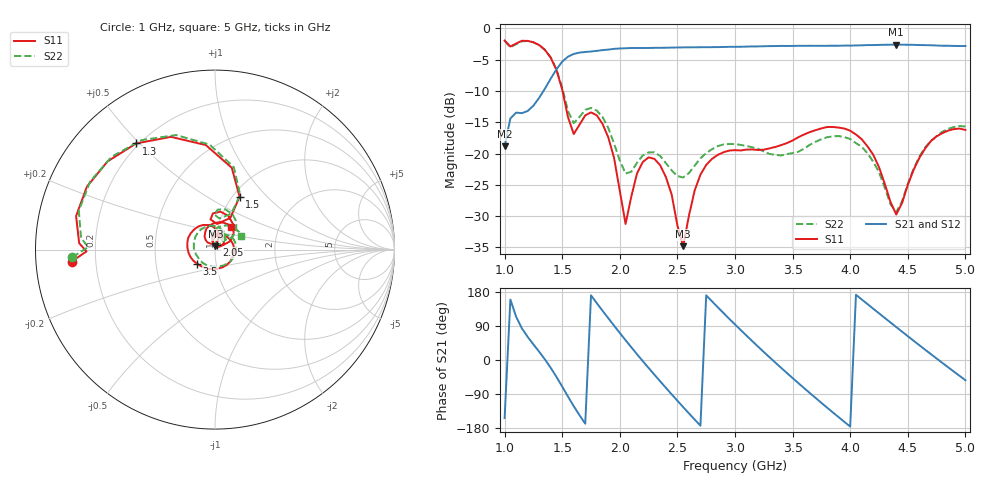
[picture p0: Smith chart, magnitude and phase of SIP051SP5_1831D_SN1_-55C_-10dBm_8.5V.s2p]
# GHz  S  dB  R  50
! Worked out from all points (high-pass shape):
!   81 points, 1 GHz to 5 GHz, reference 50 ohm
!   highest |S21| = -2.60 dB at 4.4 GHz (marker M1); lowest = -18.8 dB at 1 GHz (marker M2)
!   |S21| within 3 dB of the highest: 1.488 GHz to end of sweep
!   lowest |S11| = -34.8 dB at 2.55 GHz (marker M3), VSWR 1.04, Z = 50.2 + j1.82 ohm
!   |S11| at or under -10 dB: 1.503 GHz to end of sweep
!   |S22| runs from -29.4 to -2.0 dB; largest |S21 - S12| = 0.0021
!   S11 on the Smith chart (normalised r, x): 1 GHz: 0.11, -0.04; 1.3 GHz: 0.19, +0.49; 1.5 GHz: 1.08, +0.71; 2.05 GHz: 1.02, +0.05; 3.5 GHz: 0.81, -0.13; 5 GHz: 1.16, +0.30
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1  -1.93 -175.2  -18.83 -153.3  -18.81 -153.1  -1.98 -176.9
1.1  -2.41 177.3  -13.46 114.1  -13.45 114.0  -2.51 175.1
1.3  -2.65 126.6  -11.09 21.9  -11.10 21.7  -2.68 123.9
1.5  -9.76 65.1  -5.32 -70.1  -5.31 -70.1  -9.47 65.3
1.6  -16.87 85.6  -4.08 -121.8  -4.07 -121.7  -15.14 82.1
1.7  -13.89 93.3  -3.76 -168.1  -3.77 -168.0  -13.01 86.0
1.9  -17.40 39.9  -3.38 110.3  -3.37 110.4  -15.90 42.4
2.05  -31.24 72.2  -3.17 52.3  -3.17 52.3  -23.19 51.3
2.2  -21.33 91.7  -3.13 -3.1  -3.13 -3.1  -20.29 67.8
2.35  -21.85 52.2  -3.10 -56.1  -3.10 -56.0  -20.37 48.4
2.55  -34.79 83.7  -3.03 -124.2  -3.03 -124.2  -23.81 53.5
2.75  -21.81 79.3  -3.01 170.6  -3.01 170.7  -19.91 53.8
3  -19.45 -2.3  -2.94 93.8  -2.94 93.8  -18.49 10.8
3.25  -19.37 -81.6  -2.85 21.2  -2.86 21.2  -19.65 -48.5
3.5  -17.91 -141.9  -2.80 -47.7  -2.79 -47.7  -19.93 -132.5
3.7  -16.25 176.3  -2.79 -100.2  -2.79 -100.2  -18.10 161.6
4  -16.35 115.6  -2.75 -175.7  -2.75 -175.7  -17.67 86.9
4.15  -18.83 86.8  -2.67 147.6  -2.67 147.5  -19.95 56.7
4.35  -27.73 77.0  -2.61 99.0  -2.62 99.0  -28.09 51.4
4.4  -29.74 99.2  -2.60 86.9  -2.60 86.9  -29.37 72.7
4.7  -18.01 112.2  -2.69 15.6  -2.69 15.6  -18.00 82.5
5  -16.21 53.5  -2.81 -53.4  -2.82 -53.4  -15.68 27.1
